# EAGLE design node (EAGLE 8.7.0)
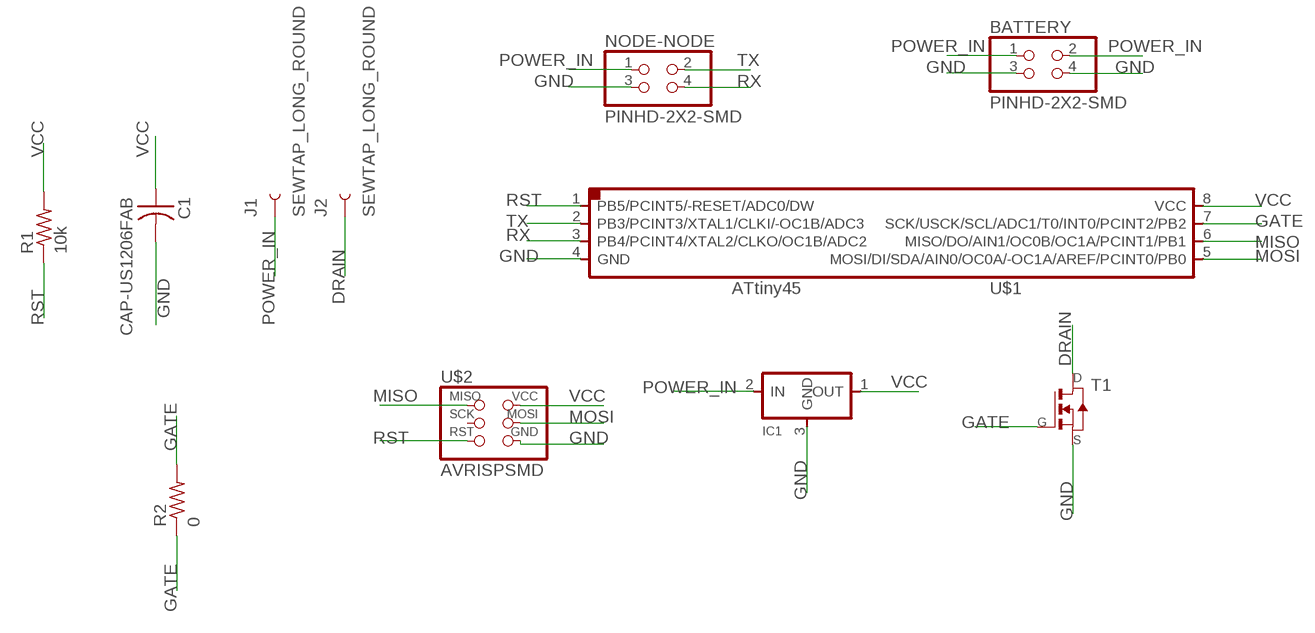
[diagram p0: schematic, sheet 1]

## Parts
BATTERY  PINHD-2X2-SMD  [2X02SMD]
C1  CAP-US1206FAB  [C1206FAB]
IC1  REGULATORSOT23  [SOT23]
J1  SEWTAP_LONG_ROUND  [PETAL-LONG-2]
J2  SEWTAP_LONG_ROUND  [PETAL-LONG-2]
NODE-NODE  PINHD-2X2-SMD  [2X02SMD]
R1  10k  RES-US1206FAB  [R1206FAB]
R2  0  RES-US1206FAB  [R1206FAB]
T1  NMOSFETSOT23  [SOT-23]
U$1  ATTINY45SI  [SOIC8]
U$2  AVRISPSMD  [2X03SMD]

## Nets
DRAIN: J2.1 T1.1(D)
GATE: R2.1 R2.2 T1.3(G) U$1.7(SCK/USCK/SCL/ADC1/T0/INT0/PCINT2/PB2)
GND: BATTERY.3 BATTERY.4 C1.2 IC1.3(GND) NODE-NODE.3 T1.2(S) U$1.4(GND) U$2.6(GND)
MISO: U$1.6(MISO/DO/AIN1/OC0B/OC1A/PCINT1/PB1) U$2.1(MISO)
MOSI: U$1.5(MOSI/DI/SDA/AIN0/OC0A/-OC1A/AREF/PCINT0/PB0) U$2.4(MOSI)
POWER_IN: BATTERY.1 BATTERY.2 IC1.2(IN) J1.1 NODE-NODE.1
RST: R1.1 U$1.1(PB5/PCINT5/-RESET/ADC0/DW) U$2.5(RST)
RX: NODE-NODE.4 U$1.3(PB4/PCINT4/XTAL2/CLKO/OC1B/ADC2)
TX: NODE-NODE.2 U$1.2(PB3/PCINT3/XTAL1/CLKI/-OC1B/ADC3)
VCC: C1.1 IC1.1(OUT) R1.2 U$1.8(VCC) U$2.2(VCC)
Unconnected: U$2.3(SCK)

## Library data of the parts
BATTERY NODE-NODE = fab:PINHD-2X2-SMD
C1 = fab:CAP-US
IC1 = fab:REGULATOR
J1 J2 = LilyPad-Wearables:SEWTAP: SparkFun LilyPad Sew Taps
R1 R2 = fab:RES-US: Resistor (US Symbol)
T1 = fab:NMOSFET: MOS FET
U$1 = fab:ATTINY45
U$2 = fab:AVRISP

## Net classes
0 default: width 0.4 mm, drill 0.4 mm, clearance 0.4 mm

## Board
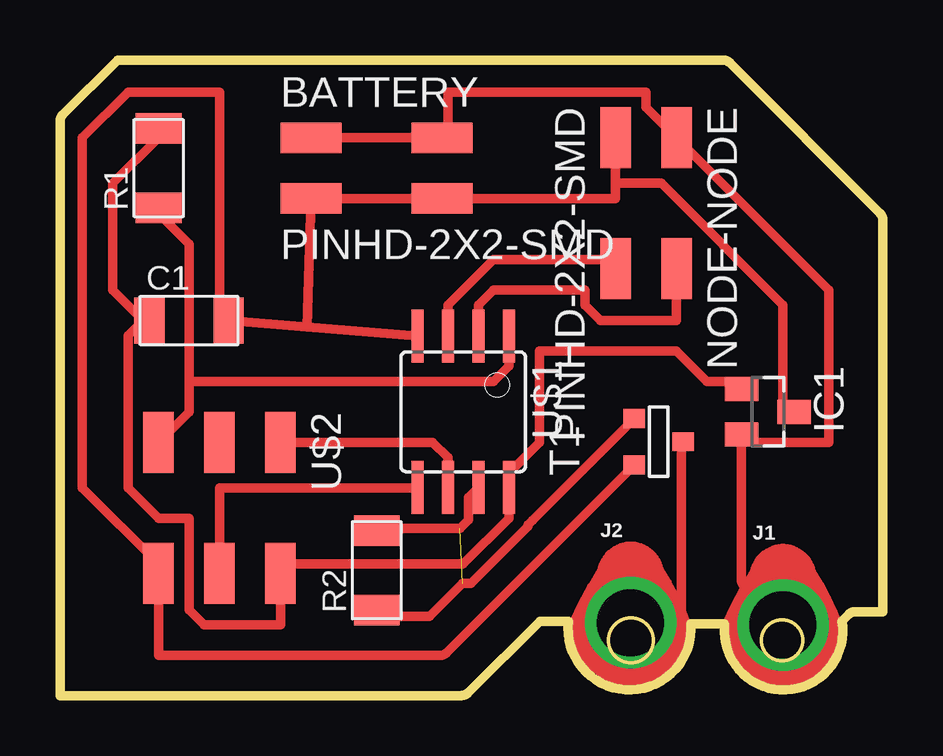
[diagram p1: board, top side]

Size 34.3 x 26.5 mm. Coordinates in mm from the lower left corner, seen from the top.
Outline: 27.7,2.9 arc194 32.6,3.1 32.88,3.38 arc-45 33.17,3.5 34.3,3.5 34.3,19.83 arc45 34.18,20.12 27.92,26.38 arc45 27.63,26.5 2.4,26.5 0.12,24.22 arc45 0,23.93 0,0 16.73,0 arc45 17.02,0.12 20,3.1 21.2,3.1 arc191 26.3,3 27.7,3
Outline: circle at 30.1,2.3 radius 0.85
Outline: circle at 23.8,2.3 radius 0.92
Copper layers (1*16): Top 0.035mm / dielectric 1.5mm / Bottom 0.035mm
Design rules "default *": minimum track width 0.4mm, minimum drill 0.35mm, track to track 0.4mm, track to pad 0.4mm, pad to pad 0.4mm, via to via 0.4mm, smd to smd 6mil, copper to edge 0.4mm, drill to drill 6mil, minimum pad ring 10mil, minimum via ring 8mil, stop-mask expansion 4mil, vias tented up to drill 0mil, thermal gap 10mil

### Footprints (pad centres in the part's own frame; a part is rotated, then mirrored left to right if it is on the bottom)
2X02SMD = smd 2.54 x 1.27: 1 -2.54,1.27; 2 2.92,1.27; 3 -2.54,-1.27; 4 2.92,-1.27
C1206FAB = smd 1.27 x 1.905: 1 -1.651,0; 2 1.651,0
SOT23 = smd 1 x 1.4: 1 -0.95,-1.1; 2 0.95,-1.1; 3 0,1.1
PETAL-LONG-2 = drill 2.794: 1 0,0
R1206FAB = smd 1.27 x 1.905: 1 -1.651,0; 2 1.651,0
SOT-23 = smd 0.787 x 0.889: 1 0.025,-1.016; 2 -0.94,1.016; 3 0.991,1.016
SOIC8 = smd 0.5 x 2.2: 1 -1.905,-3.154; 2 -0.645,-3.154; 3 0.625,-3.154; 4 1.895,-3.154; 5 1.905,3.154; 6 0.635,3.154; 7 -0.635,3.154; 8 -1.905,3.154
2X03SMD = smd 2.54 x 1.27: 1 -2.54,2.54; 2 2.92,2.54; 3 -2.54,0; 4 2.92,0; 5 -2.54,-2.54; 6 2.92,-2.54

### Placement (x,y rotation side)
BATTERY  13,21.99 0 top
C1  5.38,15.64 0 top
IC1  29.51,11.83 270 top
J1  30.14,2.94 0 top
J2  23.79,3.04 0 top
NODE-NODE  24.43,20.72 270 top
R1  4.11,21.99 90 top
R2  13.21,5.22 90 top
T1  24.96,10.56 90 top
U$1  16.81,11.83 180 top
U$2  6.65,8.02 270 top

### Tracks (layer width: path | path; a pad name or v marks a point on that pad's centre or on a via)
DRAIN
  Top 0.4: T1.1 25.9,10.58 25.9,3.44 arc-90 25.5,3.04 J2.1
GATE  (1 unrouted)
  Top 0.4: R2.1 13.36,3.42 arc45 13.65,3.3 15.4,3.3 16.78,4.68 17.14,4.68 19.52,7.05 19.52,7.12 19.7,7.3 T1.3 | U$1.7 17.03,8.26 17.03,7.33 16.67,6.98 13.32,6.98 R2.2
GND
  Top 0.4: 7.29,15.64 C1.2 | 14.91,15.01 U$1.4 10.31,15.37 | 15.54,20.72 BATTERY.4 | 23.16,21.35 25.07,21.35 30.14,16.27 30.14,11.83 IC1.3 | NODE-NODE.3 23.16,21.35 | BATTERY.4 23.16,20.72 23.16,21.35 | C1.2 6.65,15.64 6.65,25.16 2.84,25.16 0.94,23.26 0.94,8.66 4.11,5.48 U$2.6 4.11,1.67 15.83,1.67 arc45 16.11,1.79 T1.2 | C1.2 10.31,15.37 | 10.31,15.37 BATTERY.3 BATTERY.4
MISO
  Top 0.4: U$1.6 16.18,9.93 15.54,10.56 U$2.1
MOSI
  Top 0.4: U$2.4 6.65,8.66 14.91,8.66 U$1.5
POWER_IN
  Top 0.4: 28.24,10.56 IC1.2 | BATTERY.1 BATTERY.2 16.18,23.26 16.18,25.16 24.43,25.16 24.43,24.53 NODE-NODE.1 32.05,16.91 32.05,10.56 28.88,10.56 IC1.2 | IC1.2 28.41,4.84 arc45 28.53,4.55 J1.1
RST
  Top 0.4: 5.38,13.1 5.38,11.83 U$2.5 | 5.38,13.1 5.38,18.81 4.11,20.08 R1.1 | U$1.1 18.71,13.74 18.08,13.1 5.38,13.1
RX
  Top 0.4: U$1.3 16.18,15.01 16.18,16.27 18.08,18.18 23.16,18.18 NODE-NODE.4
TX
  Top 0.4: NODE-NODE.2 25.7,15.64 22.53,15.64 21.89,16.27 21.89,16.91 18.08,16.91 17.45,16.27 17.45,15.01 U$1.2
VCC
  Top 0.4: 3.47,15.64 2.21,16.91 2.21,21.35 4.11,23.26 R1.2 | IC1.1 28.24,13.1 26.97,13.1 25.7,14.37 19.98,14.37 19.98,10.56 18.71,9.29 U$1.8 18.71,7.39 16.81,5.48 9.19,5.48 U$2.2 9.19,2.94 6.01,2.94 5.38,3.57 5.38,7.39 4.11,7.39 2.84,8.66 2.84,15.01 3.47,15.64 | 3.47,15.64 C1.1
